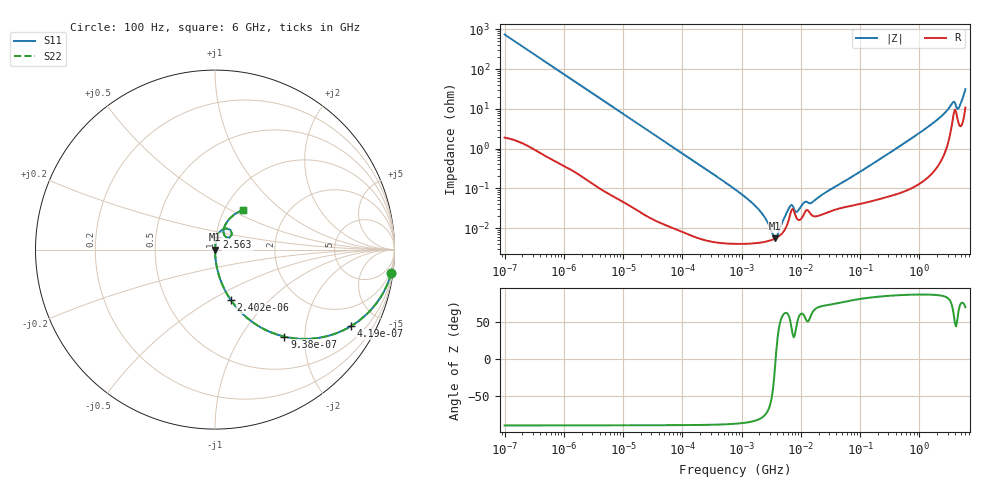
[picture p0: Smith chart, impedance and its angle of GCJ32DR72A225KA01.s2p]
!Murata Part Number: GCJ32DR72A225KA01
!These Parameters are Measured in Series Mode Connection
!Data Generated on Mar 13, 2026
!  o--ll--o
!Port1  Port2
!  o------o
!Operation Temp=25[degC], DC Bias Voltage=0[V]
!Freq. Start=100[Hz] Stop=6[GHz] 401[Steps]
# Hz S RI R 50
!Freq.(Hz) S11(Real) S11(Imag) S21(Real) S21(Imag) S12(Real) S12(Imag) S22(Real) S22(Imag)
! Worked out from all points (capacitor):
!   401 points, 100 Hz to 6 GHz, reference 50 ohm
!   read as one part in series: C = 2.15 uF near 109 Hz
!   lowest |Z| = 5.52 mohm at 3.712 MHz (marker M1)
!   series resonance near 3.762 MHz, so ESL is about 830 pH
!   S11 on the Smith chart (normalised r, x): 100 Hz: 1, -15; 419 Hz: 1.01, -3.54; 938 Hz: 1.01, -1.59; 2.402 kHz: 1.00, -0.62; 2.563 GHz: 1.01, +0.15; 6 GHz: 1.21, +0.59
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100  0.9817 -0.1327  0.0183 0.1327  0.0183 0.1327  0.9817 -0.1327
224  0.9154 -0.2763  0.0846 0.2763  0.0846 0.2763  0.9154 -0.2763
419  0.7573 -0.4266  0.2427 0.4266  0.2427 0.4266  0.7573 -0.4266
938  0.3865 -0.4845  0.6135 0.4845  0.6135 0.4845  0.3865 -0.4845
2008  0.1225 -0.3252  0.8775 0.3252  0.8775 0.3252  0.1225 -0.3252
2402  0.0893 -0.2825  0.9107 0.2825  0.9107 0.2825  0.0893 -0.2825
7695  0.00994 -0.0963  0.9901 0.0963  0.9901 0.0963  0.00994 -0.0963
40335  0.000488 -0.0187  0.9995 0.0187  0.9995 0.0187  0.000488 -0.0187
774597  4.08e-05 -0.000941  1 0.000941  1 0.000941  4.08e-05 -0.000941
1813585  4.19e-05 -0.000325  1 0.000325  1 0.000325  4.19e-05 -0.000325
3103719  4.91e-05 -8.1e-05  1 8.1e-05  1 8.1e-05  4.91e-05 -8.1e-05
3712478  5.49e-05 -5.6e-06  0.9999 5.6e-06  0.9999 5.6e-06  5.49e-05 -5.6e-06
4440638  6.53e-05 7.35e-05  0.9999 -7.35e-05  0.9999 -7.35e-05  6.53e-05 7.35e-05
6644369  0.000224 0.000282  0.9998 -0.000282  0.9998 -0.000282  0.000224 0.000282
8692127  0.000169 0.000197  0.9998 -0.000197  0.9998 -0.000197  0.000169 0.000197
1.137099e7  0.000228 0.000374  0.9998 -0.000374  0.9998 -0.000374  0.000228 0.000374
1.555665e7  0.000207 0.000392  0.9998 -0.000392  0.9998 -0.000392  0.000207 0.000392
3.124326e8  0.000685 0.00768  0.9993 -0.00768  0.9993 -0.00768  0.000685 0.00768
2.562649e9  0.0116 0.0715  0.9884 -0.0715  0.9884 -0.0715  0.0116 0.0715
3.666503e9  0.0656 0.1176  0.9344 -0.1176  0.9344 -0.1176  0.0656 0.1176
4.586474e9  0.0498 0.0837  0.9502 -0.0837  0.9502 -0.0837  0.0498 0.0837
6e9  0.1556 0.2233  0.8444 -0.2233  0.8444 -0.2233  0.1556 0.2233
